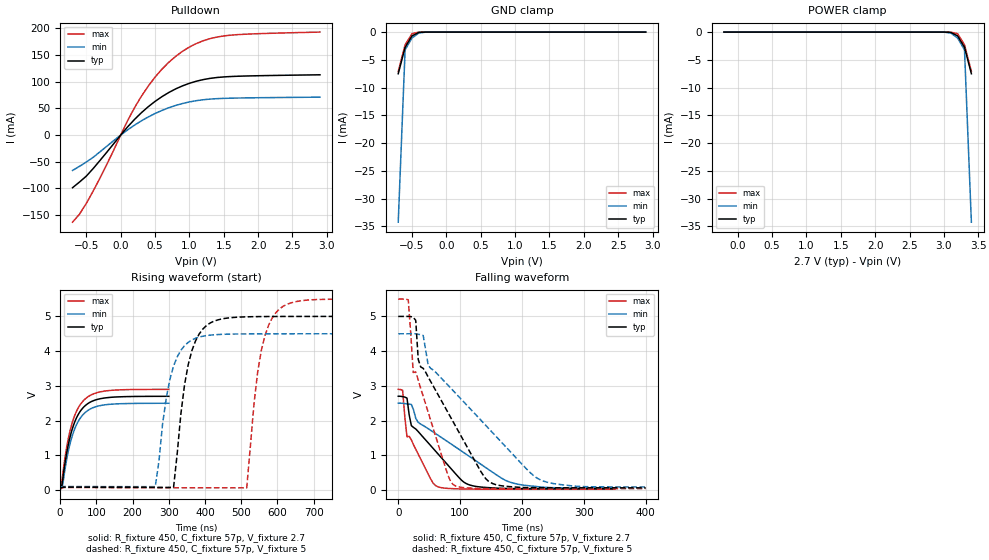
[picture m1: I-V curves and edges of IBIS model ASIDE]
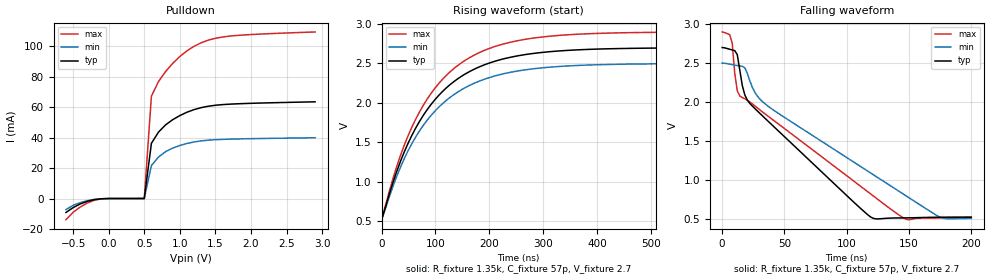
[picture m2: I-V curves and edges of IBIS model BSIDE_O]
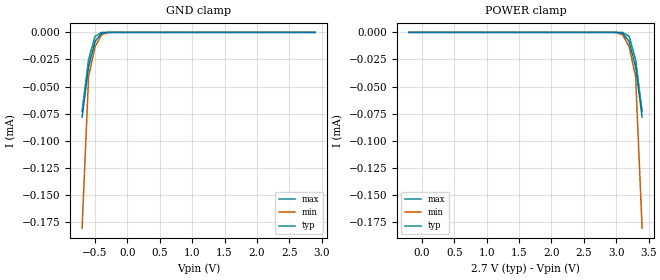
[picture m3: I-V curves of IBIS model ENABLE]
[IBIS Ver]   3.2
[Comment Char]   |_char
| VDD nom: 2.7v, min: 2.5v, max:2.9v
[File name]   pca9507_a_2_7.ibs
[File Rev]   1
[Date]   Sep 19, 2008 3:12:36 PM
[Source]
Generated using IBISToolkit at NXP Tempe by Seshadri Venkataramanan
[Notes]
[Disclaimer]
(C) Copyright 2007 NXP Semiconductors
All rights reserved
NXP Semiconductors (NXP) does not warrant that this model and any other
accompanying information (Model) accurately or fully represents the
operating characteristics and specifications of the semiconductor
products to which the Model relates.  Moreover, the Model is furnished
on an "as is" and with "all faults" basis, and without support or
warranty of any kind.  NXP disclaims all warranties, whether expressed
or implied or statutory, including without limitation all implied
warranties of non-infringement, merchantability and fitness for any
purpose, and those arising from a course of dealing or usage of trade.
NXP does not convey any license under its or any third party's patents,
copyrights or other intellectual property or proprietary rights.
You and your company assume any and all risks and liability arising out
of the application or use of the Model.
In no event shall NXP be liable for any direct, indirect, special,
consequential or incidental damages, however caused, whether in
warranty, contract or tort (including negligence), strict liability or
other legal theory, including, without limitation, for lost profits,
business interruption, or corruption or loss of data or information,
arising out of or in connection with the use of or the inability to use
the Model, even if NXP has been advised of the possibility of such
damages.
NXP provides the Model as a courtesy to our customers. You and your
company shall not distribute, convey, sell, or give the Model to anyone
else without receiving prior written permission from NXP.
NXP reserves the right to make changes without notice to the Model to
improve reliability, function, or design.
Please be aware that your receipt and subsequent use of the Model shall
serve as acceptance of these terms and conditions.  If you do not
accept these terms, return or destroy the Model immediately.
[Copyright]
2008
| SO8
[Component]   PCA9507D
Si_location Pin
Timing_location Pin
[Manufacturer]   NXP
[Package]
R_pkg   4.81E-02   4.14E-02   5.47E-02
L_pkg   1.88n   1.54n   2.21n
C_pkg   4.49E-13   4.17E-13   4.81E-13
[Pin] signal_name   model_name   R_pin   L_pin   C_pin
1   VCCA   POWER   5.47E-02  2.21E-09  4.81E-13
2   SCLA   ASIDE   4.14E-02  1.54E-09  4.20E-13
3   SDAA   ASIDE   4.14E-02  1.55E-09  4.20E-13
4   GND   GND   5.47E-02  2.21E-09  4.80E-13
5   EN   ENABLE   5.47E-02  2.21E-09  4.78E-13
6   SDAB   BSIDE_I/O   4.14E-02  1.55E-09  4.17E-13
7   SCLB   BSIDE_I/O   4.14E-02  1.54E-09  4.17E-13
8   VCCB   POWER   5.47E-02  2.21E-09  4.79E-13
| TSSOP8
[Component]   PCA9507AD
Si_location Pin
Timing_location Pin
[Manufacturer]   NXP
[Package]
R_pkg   33.7m   30.1m   37.3m
L_pkg   1.74n   1.67n   1.81n
C_pkg   0.428p   0.422p   0.434p
[Pin] signal_name   model_name   R_pin   L_pin   C_pin
1   VCCA   POWER   37.3m   1.81nH   0.428pF
2   SCLA   ASIDE   30.1m   1.67nH   0.422pF
3   SDAA   ASIDE   30.1m   1.67nH   0.428pF
4   GND   GND   37.3m   1.81nH   0.434pF
5   EN   ENABLE   37.3m   1.81nH   0.428pF
6   SDAB   BSIDE_I/O   30.1m   1.67nH   0.422pF
7   SCLB   BSIDE_I/O   30.1m   1.67nH   0.428pF
8   VCCB   POWER   37.3m   1.81nH   0.434pF
[Model Selector]   BSIDE_I/O
BSIDE_I   Bside as Input
BSIDE_O   Bside as Output
| Models and submodels in the file (4): ASIDE (I/O_open_drain), BSIDE_O (Open_drain), ENABLE (Input), BSIDE_I (Input)
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[Model]   ASIDE
Model_type I/O_open_drain
Vinh=1.89
Vinl=0.81
Vref=2.7
Vmeas=1.35
Rref=450
Cref=57p
C_comp   5.2p   5p   5.4p
[Temperature Range] 27   85   -40
[Voltage Range]   2.7   2.5   2.9
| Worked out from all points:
|   slope of the pulldown table from 0 to 0.405 V, typ, clamps not added: 7.55 ohm
|   GND clamp passes 1 mA (typ) near -0.52 V on its own axis
|   falling waveform, R_fixture 450, C_fixture 57p, V_fixture 2.7: 20-80 % time 69.9ns typ, 120ns min, 34.9ns max; typ from 2.7 V to 0.038 V
|   falling waveform, R_fixture 450, C_fixture 57p, V_fixture 5: 20-80 % time 85.9ns typ, 140ns min, 47.2ns max; typ from 5 V to 0.061 V
|   rising waveform, R_fixture 450, C_fixture 57p, V_fixture 2.7: 20-80 % time 39ns typ, 39.2ns min, 38.9ns max; typ from 0.038 V to 2.7 V
|   rising waveform, R_fixture 450, C_fixture 57p, V_fixture 5: 20-80 % time 40.5ns typ, 40.9ns min, 40.5ns max; typ from 0.061 V to 5 V
[Pulldown]
-700mV    -98.57mA   -66.12mA   -163.2mA
-600mV    -88.08mA   -58.57mA   -148.3mA
-400mV    -62.69mA   -41.65mA   -104.9mA
-200mV    -31.79mA   -20.67mA   -54.57mA
100mV     15.26mA    9.678mA    26.77mA
300mV     41.78mA    26.67mA    72.52mA
500mV     63.17mA    40.5mA     108.6mA
800mV     86.61mA    55.63mA    147.6mA
1.1V      101mA      64.57mA    171.6mA
1.4V      108mA      68.38mA    183.8mA
1.8V      110.8mA    69.76mA    189.1mA
2.9V      113.1mA    71.21mA    193.2mA
[GND Clamp]
-700mV    -7.503mA   -34.23mA   -7.098mA
-600mV    -2.746mA   -3.201mA   -2.289mA
-500mV    -684.9uA   -1.067mA   -291.2uA
-400mV    -56.26uA   -166.1uA   -7.856uA
-300mV    -1.512uA   -7.935uA   -82.32nA
2.9V      196.5pA    374pA      180.4pA
[POWER Clamp]
-200mV    196.5pA    374pA      180.4pA
3V        -1.508uA   -7.926uA   -81.85nA
3.1V      -56.15uA   -166uA     -7.816uA
3.2V      -684.2uA   -1.066mA   -290.3uA
3.3V      -2.744mA   -3.2mA     -2.285mA
3.4V      -7.501mA   -34.23mA   -7.091mA
[Falling Waveform]
R_fixture=450
C_fixture=57p
V_fixture=2.7
V_fixture_min=2.5
V_fixture_max=2.9
0s        2.7V       2.5V       2.9V
7.071ns   2.689V     2.497V     2.874V
14.14ns   2.648V     2.48V      1.532V
21.21ns   1.853V     2.464V     1.443V
31.82ns   1.692V     1.956V     1.052V
56.57ns   1.194V     1.669V     191.8mV
63.64ns   1.052V     1.585V     96.1mV
109.6ns   187.4mV    1.032V     25.73mV
183.8ns   40.54mV    207.7mV    23.16mV
350ns     37.88mV    55.76mV    23.08mV
[Falling Waveform]
R_fixture=450
C_fixture=57p
V_fixture=5
V_fixture_min=4.5
V_fixture_max=5.5
0s        5V         4.5V       5.5V
16.16ns   5V         4.5V       5.477V
24.24ns   4.976V     4.5V       3.385V
28.28ns   4.886V     4.499V     3.401V
36.36ns   3.543V     4.471V     2.919V
48.48ns   3.251V     3.591V     2.235V
88.89ns   1.96V      2.859V     155.3mV
153.5ns   178.3mV    1.631V     39.97mV
234.3ns   62.63mV    258.8mV    39.21mV
400ns     61.43mV    86.93mV    39.15mV
[Rising Waveform]
R_fixture=450
C_fixture=57p
V_fixture=2.7
V_fixture_min=2.5
V_fixture_max=2.9
0s        37.78mV    55.16mV    23.07mV
3.03ns    40.8mV     55.4mV     77.58mV
6.061ns   212.2mV    86.68mV    354.5mV
18.18ns   1.073V     891.5mV    1.242V
30.3ns    1.643V     1.45V      1.827V
48.48ns   2.146V     1.949V     2.336V
69.7ns    2.434V     2.236V     2.627V
93.94ns   2.579V     2.382V     2.775V
130.3ns   2.659V     2.46V      2.858V
300ns     2.698V     2.498V     2.897V
[Rising Waveform]
R_fixture=450
C_fixture=57p
V_fixture=5
V_fixture_min=4.5
V_fixture_max=5.5
0s        61.32mV    86.34mV    39.12mV
262.6ns   74.93mV    94.31mV    62.76mV
292.9ns   74.46mV    2.642V     62.1mV
313.1ns   74.36mV    3.569V     61.88mV
343.4ns   3.029V     4.156V     61.72mV
373.7ns   4.292V     4.37V      61.64mV
515.2ns   4.987V     4.495V     61.51mV
545.5ns   4.993V     4.496V     3.404V
596ns     4.997V     4.498V     5.111V
1us       4.999V     4.499V     5.498V
[Ramp]
R_load=450
dV/dt_r   1.608E-5/1.001E-8   9.245E-6/2.282E-9   3.355E-5/1.172E-7
dV/dt_f   1.707E-5/1.750E-7   7.931E-6/1.569E-7   4.331E-5/1.970E-7
|[End   ASIDE
[Model]   BSIDE_O
Model_type Open_drain
Vref=2.7
Vmeas=1.35
Rref=1.35k
Cref=57p
C_comp   4.8p   4.6p   5p
[Temperature Range] 27   85   -40
[Voltage Range]   2.7   2.5   2.9
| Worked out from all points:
|   slope of the pulldown table from 0 to 0.405 V, typ, clamps not added: 29.4 kohm
|   falling waveform, R_fixture 1.35k, C_fixture 57p, V_fixture 2.7: 20-80 % time 73.9ns typ, 110ns min, 95.1ns max; typ from 2.7 V to 0.52 V
|   rising waveform, R_fixture 1.35k, C_fixture 57p, V_fixture 2.7: 20-80 % time 114ns typ, 114ns min, 113ns max; typ from 0.516 V to 2.7 V
[Pulldown]
-600mV    -9.148mA   -7.265mA   -13.9mA
-400mV    -3.558mA   -2.7mA     -5.599mA
-200mV    -716.2uA   -567.5uA   -1.091mA
500mV     10.52uA    32.98uA    4.183uA
600mV     36.23mA    21.62mA    67.15mA
700mV     43.61mA    27.25mA    76.82mA
800mV     48.39mA    30.79mA    83.39mA
900mV     51.77mA    33.12mA    88.78mA
1.1V      56.66mA    36.15mA    96.99mA
1.3V      59.67mA    37.84mA    102.3mA
1.6V      61.66mA    38.82mA    106mA
2.9V      63.48mA    39.9mA     109.3mA
[Falling Waveform]
R_fixture=1.35k
C_fixture=57p
V_fixture=2.7
V_fixture_min=2.5
V_fixture_max=2.9
0s        2.7V       2.5V       2.9V
8.081ns   2.669V     2.48V      2.752V
12.12ns   2.609V     2.469V     2.144V
14.14ns   2.41V      2.463V     2.078V
22.22ns   1.981V     2.271V     2V
36.36ns   1.761V     1.952V     1.823V
119.2ns   521.8mV    1.087V     818.3mV
147.5ns   510.4mV    795.1mV    493.5mV
175.8ns   519mV      513.9mV    509.8mV
200ns     519.6mV    503.6mV    515.8mV
[Rising Waveform]
R_fixture=1.35k
C_fixture=57p
V_fixture=2.7
V_fixture_min=2.5
V_fixture_max=2.9
0s        516.5mV    517.8mV    516.9mV
21.21ns   990.5mV    941.7mV    1.041V
35.35ns   1.262V     1.188V     1.338V
56.57ns   1.591V     1.487V     1.696V
77.78ns   1.844V     1.717V     1.972V
120.2ns   2.189V     2.031V     2.348V
176.8ns   2.441V     2.262V     2.621V
240.4ns   2.579V     2.388V     2.77V
332.3ns   2.659V     2.462V     2.856V
700ns     2.699V     2.499V     2.899V
[Ramp]
R_load=1350
dV/dt_r   1.309E+0/8.275E-9   1.307E+0/7.928E-9   1.309E+0/7.975E-9
dV/dt_f   1.308E+0/6.940E-8   1.305E+0/1.219E-7   1.310E+0/7.434E-8
|[End   BSIDE_O
[Model]   ENABLE
Model_type Input
Vinh=1.89
Vinl=0.81
C_comp   1.7p   1.5p   1.9p
[Temperature Range] 27   85   -40
[Voltage Range]   2.7   2.5   2.9
[GND Clamp]
-700mV    -78.2uA    -180.8uA   -72.93uA
-600mV    -31.83uA   -40.84uA   -25.27uA
-500mV    -8.452uA   -13.3uA    -3.68uA
-400mV    -758.4nA   -2.213uA   -96.83nA
-300mV    -18.6nA    -106.4nA   -805pA
-200mV    -273.4pA   -2.436nA   -5.553pA
2.9V      5.862pA    7.156pA    5.8pA
[POWER Clamp]
-200mV    5.862pA    7.156pA    5.8pA
2.9V      -273.4pA   -2.436nA   -5.553pA
3V        -18.6nA    -106.4nA   -805pA
3.1V      -758.4nA   -2.213uA   -96.83nA
3.2V      -8.452uA   -13.3uA    -3.68uA
3.3V      -31.83uA   -40.84uA   -25.27uA
3.4V      -78.2uA    -180.8uA   -72.93uA
